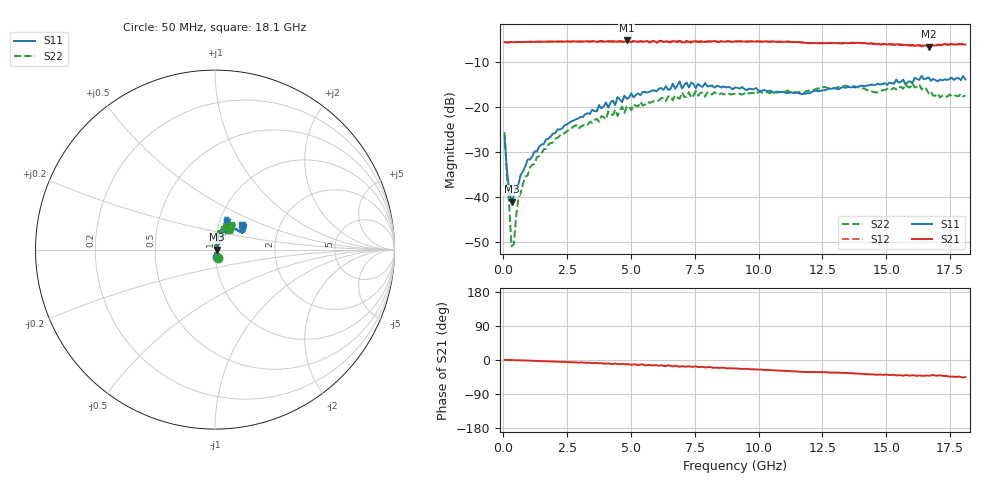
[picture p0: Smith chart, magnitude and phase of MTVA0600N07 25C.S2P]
! Network Analyzer HP8720D.06.14 Serial No. US36140669
!  6 Jul 2005  09:11:06
! Frequency  S11  S21  S12  S22
# HZ  S  DB R 50
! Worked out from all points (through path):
!   201 points, 50 MHz to 18.1 GHz, reference 50 ohm
!   highest |S21| = -5.16 dB at 4.833 GHz (marker M1); lowest = -6.5 dB at 16.66 GHz (marker M2)
!   group delay of S21, straight-line fit = 7.26 ps
!   lowest |S11| = -41.1 dB at 320.8 MHz (marker M3), VSWR 1.02, Z = 50.9 - j0.112 ohm
!   |S11| at or under -10 dB: start of sweep to end of sweep
!   |S22| runs from -51.0 to -14.7 dB; largest |S21 - S12| = 0.024
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5e7  -26.78 -72.4  -5.53 0.3  -5.54 0.3  -25.65 -70.2
1.4025e8  -34.06 -58.3  -5.61 -0.0  -5.59 0.0  -35.30 -92.2
2.305e8  -38.53 -35.8  -5.54 -0.2  -5.54 -0.1  -41.73 -106.0
3.2075e8  -41.11 -7.1  -5.51 -0.1  -5.53 -0.1  -50.99 -133.8
4.11e8  -39.76 16.9  -5.55 -0.6  -5.54 -0.6  -50.57 129.9
5.915e8  -37.20 42.1  -5.50 -0.6  -5.54 -0.7  -40.30 98.7
1.04275e9  -31.68 57.5  -5.45 -1.9  -5.46 -1.8  -33.46 82.4
2.30625e9  -24.77 56.7  -5.42 -4.8  -5.41 -4.9  -25.82 77.5
3.1185e9  -22.21 61.5  -5.40 -6.4  -5.43 -6.9  -24.05 80.7
4.47225e9  -17.78 58.7  -5.46 -10.5  -5.31 -9.7  -21.95 81.3
4.83325e9  -18.16 67.7  -5.16 -11.3  -5.37 -11.9  -19.90 70.5
6.09675e9  -15.87 63.9  -5.35 -14.9  -5.27 -14.7  -18.52 71.9
6.7285e9  -15.93 70.7  -5.37 -14.5  -5.61 -15.3  -17.40 67.0
6.909e9  -14.28 68.5  -5.23 -18.0  -5.34 -16.4  -18.16 65.9
6.99925e9  -15.89 68.4  -5.49 -16.1  -5.62 -17.9  -16.73 67.5
7.17975e9  -14.54 72.7  -5.25 -17.5  -5.48 -16.4  -17.77 62.5
9.075e9  -15.62 67.3  -5.36 -22.3  -5.34 -22.3  -17.07 61.0
1.21435e10  -16.47 51.8  -5.74 -31.6  -5.70 -31.6  -16.20 61.1
1.512175e10  -14.56 32.3  -6.06 -39.8  -5.89 -39.4  -16.10 60.7
1.602425e10  -14.75 39.1  -6.16 -40.2  -6.34 -42.3  -14.71 54.1
1.6656e10  -13.38 38.7  -6.51 -41.4  -6.37 -40.1  -16.94 46.3
1.81e10  -13.84 42.1  -6.08 -45.0  -6.25 -45.7  -17.44 54.6
